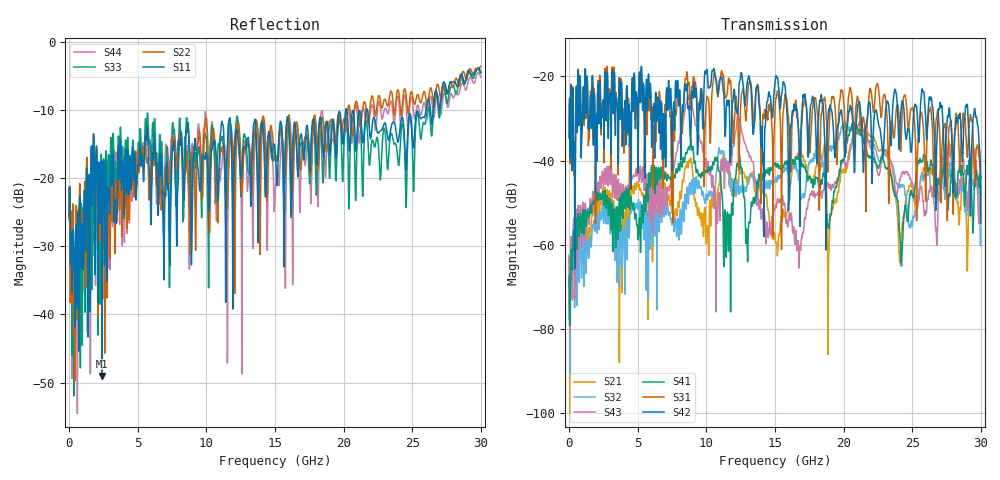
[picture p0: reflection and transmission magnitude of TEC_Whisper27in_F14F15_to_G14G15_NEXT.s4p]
! Tyco Electronics
! F14F15-G14G15_NEXT
!! PART DESCRIPTION: Whisper 27in Megtron 6 VLP-HVLP-VLP Channel Model, bulkhead 2.4mm test pts
!! MODEL DESCRIPTION: System 4-port S-parameter
!! MODEL STATUS: Measured
!! MODEL GEOMETRY: Channel Model
!! MODEL FREQUENCY RANGE: DC to 30.000 GHz in 10.000 MHz frequency steps
!! MODEL EDGE RATE LIMITATION: 12.500 ps (Using conservative 0.5/Fmax rule of thumb)
!! TIME-DOMAIN TRANSFORM CAUTIONS:
!! 1.) Do not simulate transient edge rates faster than the number listed above.  Edge rates faster than this number
!!  contain significant spectral content at frequencies above the model's highest frequency.
!! 2.) Even when simulating edge rates that are slower than the number listed above, be aware that the best time
!!  resolution possible with a direct iFFT is (1 / 2Fmax).  As a result, time resolution is typically not adequate
!!  for most time-domain simulations unless tricks such as windowing are used to minimize leakage and aliasing.
!! 3.) Because the model has a uniform frequency step, a direct iFFT will result in an impulse that that has a time
!!  length given by either (1 / Fstep) or (1 / 2Fstep), depending on the transform being used.  Care has been taken
!!  in selecting the frequency step to ensure a settled impulse response for the model.  Therefore, convolution with
!!  the model's impulse response should present no issues.  However, if directly concatenating s-parameter models
!!  in the frequency domain a user must either interpolate necessary interim frequencies or complete impulse response
!!  zero-padding.  Impulse response zero-padding is more difficult, but more accurate.
!! PORT DEFINITIONS:
!! Port  1  ----->  Side A  F14  G14  Side A  <-----  Port  2
!! Port  3  ----->  Side A  F15  G15  Side A  <-----  Port  4
! Point-to-Point link (differential)  !
! Connectors:  !
!  1: STRADA Whisper  !
! Materials:  !
!  Backplane: Megtron-6 HVLP  !
!  Daughtercard: Megtron-6 VLP  !
! Stack-up:  !
!  Backplane: 20 layers, 200mil thick  !
!  Daughtercard: 14 layers, 110mil thick  !
! Trace Length:  !
!  Backplane: 17in  !
!  Daightercards: 5in  !
! Trace Width:  !
!  Backplane: 8-13-8 mils  !
!  Daughtercards: 6-9-6 mils  !
! Geometry:  !
!  Backplane: Stripline  !
!  Daughtercards: Stripline  !
! Freq. Range: 0 GHz - 30 GHz  !
! Note1: non-mixed-mode s-parameters  !
! Note2: channel includes 2.4mm test points  !
! Touchstone data converted from IdEM dataset
# GHz S MA R 50
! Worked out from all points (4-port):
!   3000 points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, 10 MHz to 30 GHz, reference 50 ohm
!   strongest paths, dB at 10 MHz, 7.51 GHz, 15.01 GHz, 22.51 GHz, 30 GHz:
!     S42: -34.5, -34.3, -21.3, -30.6, -54.8
!     S31: -34.7, -36.1, -28.3, -22.2, -43.8
!     S41: -67.5, -44.5, -40.8, -41.7, -48.2
!     S43: -63.1, -44.3, -51.2, -43.3, -48.6
!     S32: -62.5, -55.2, -44.9, -39.5, -56.2
!     S21: -62.5, -52.3, -58.1, -37.4, -44.1
!   lowest |S11| = -49.0 dB at 2.41 GHz (marker M1), VSWR 1.01, Z = 49.9 - j0.34 ohm
!   |S11| at or under -10 dB: start of sweep to 20.16 GHz; 20.23 GHz to 21.65 GHz (1.417 GHz wide, 6.77 % of centre); 21.75 GHz to 26 GHz (4.25 GHz wide, 17.8 % of centre)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
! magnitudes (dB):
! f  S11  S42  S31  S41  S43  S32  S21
! 10 MHz  -25.5  -34.5  -34.7  -67.5  -63.1  -62.5  -62.5
! 2.41 GHz  -49.0  -28.6  -27.7  -48.6  -43.0  -51.2  -48.9
! 8.77 GHz  -15.1  -29.6  -23.2  -37.4  -24.8  -45.4  -40.0
! 15.16 GHz  -21.0  -20.3  -23.6  -41.1  -49.4  -44.7  -61.0
! 16.74 GHz  -17.6  -35.0  -34.0  -39.5  -64.4  -44.6  -38.4
! 20.1 GHz  -11.2  -38.2  -31.8  -37.7  -40.4  -30.8  -41.9
! 30 GHz  -4.4  -54.8  -43.8  -48.2  -48.6  -56.2  -44.1
